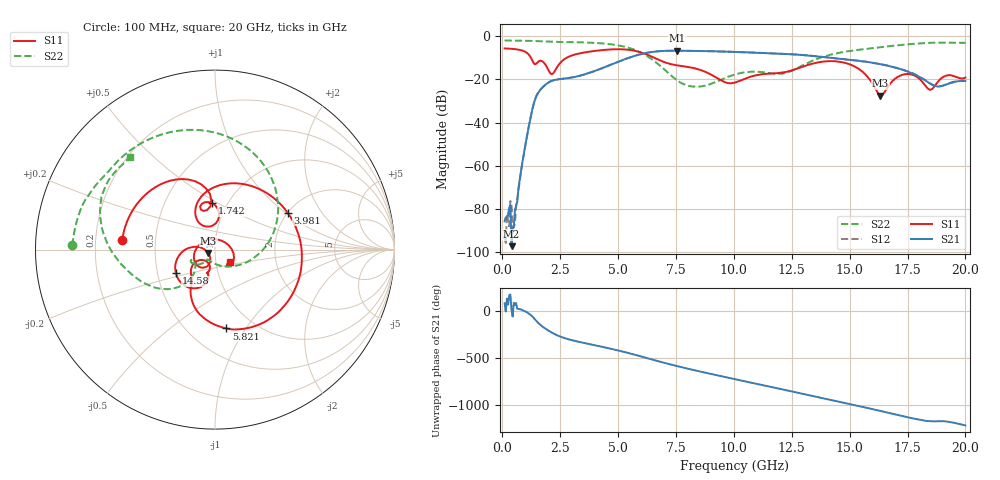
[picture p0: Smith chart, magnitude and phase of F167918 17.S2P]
!  2-Port S-parameters saved by WinCal
! VAR MeasName=S-Parameters (CALIBRATED_DATA) read from VNA (N5242A)
! VAR MeasDate=2016-11-22 10:25:36
! VAR NAME=F167918 17
! VAR FILENAME=F167918 17.S2P
! VAR DATE=2016-11-22 10:25:37
! VAR PHYS_PORTS=1,2
# Hz S DB R 50
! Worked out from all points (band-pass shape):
!   401 points, 100 MHz to 20 GHz, reference 50 ohm
!   highest |S21| = -6.74 dB at 7.562 GHz (marker M1); lowest = -97.2 dB at 398.5 MHz (marker M2)
!   |S21| within 3 dB of the highest: 5.545 GHz to 13.89 GHz (8.349 GHz wide, 85.9 % of centre)
!   lowest |S11| = -27.6 dB at 16.32 GHz (marker M3), VSWR 1.09, Z = 46.3 - j1.69 ohm
!   |S11| at or under -10 dB: 1.237 GHz to 2.78 GHz (1.544 GHz wide, 76.9 % of centre); 6.561 GHz to end of sweep
!   |S22| runs from -23.4 to -2.0 dB; largest |S21 - S12| = 0.004
!   S11 on the Smith chart (normalised r, x): 100 MHz: 0.32, +0.05; 1.742 GHz: 0.85, +0.47; 3.981 GHz: 2.00, +1.04; 5.821 GHz: 0.75, -0.82; 14.58 GHz: 0.62, -0.17; 20 GHz: 1.17, -0.16
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1e8  -5.69 174.1  -85.72 77.6  -92.25 -49.3  -2.00 178.3
3.985e8  -5.85 156.2  -97.25 7.1  -78.10 143.5  -2.04 173.5
5.975e8  -6.09 143.7  -78.56 82.4  -78.42 25.6  -2.07 170.3
1.34375e9  -12.30 96.1  -31.91 -73.7  -31.88 -74.0  -2.26 158.1
1.74175e9  -11.73 93.5  -23.70 -169.1  -23.68 -169.4  -2.43 151.9
2.13975e9  -17.61 102.5  -20.70 127.6  -20.66 127.5  -2.61 145.9
3.43325e9  -7.78 60.2  -18.08 22.7  -18.08 22.5  -2.88 122.6
3.9805e9  -6.86 27.0  -16.18 -5.8  -16.19 -5.9  -3.13 109.5
4.82625e9  -6.09 -23.8  -12.63 -51.2  -12.63 -51.3  -3.97 83.9
5.82125e9  -7.05 -81.8  -8.80 -113.6  -8.77 -113.5  -6.81 40.8
6.7665e9  -11.01 -118.8  -6.99 -178.2  -6.97 -178.2  -13.27 -13.4
7.5625e9  -13.55 -127.4  -6.74 131.2  -6.73 131.1  -20.55 -72.2
8.60725e9  -15.86 -143.5  -6.91 71.1  -6.89 71.0  -23.22 -126.6
1.005e10  -21.51 -116.4  -7.30 -7.3  -7.30 -7.2  -17.79 -139.7
1.1642e10  -17.33 -108.2  -7.95 -90.9  -7.93 -90.9  -17.20 -155.2
1.338325e10  -12.80 -112.5  -9.15 175.6  -9.10 175.8  -11.44 -132.4
1.457725e10  -11.91 -149.1  -10.49 112.7  -10.44 112.7  -7.67 -150.8
1.63185e10  -27.57 -154.2  -12.97 16.5  -12.92 17.3  -5.14 -175.4
1.67165e10  -22.62 -112.0  -13.84 -5.9  -13.85 -5.4  -4.66 179.4
1.746275e10  -17.48 -139.0  -16.23 -48.3  -16.09 -47.7  -3.84 169.0
1.875625e10  -21.85 16.5  -23.28 -93.5  -23.20 -92.9  -3.02 148.5
2e10  -19.19 -38.8  -20.71 -137.8  -20.58 -137.6  -3.11 132.5
